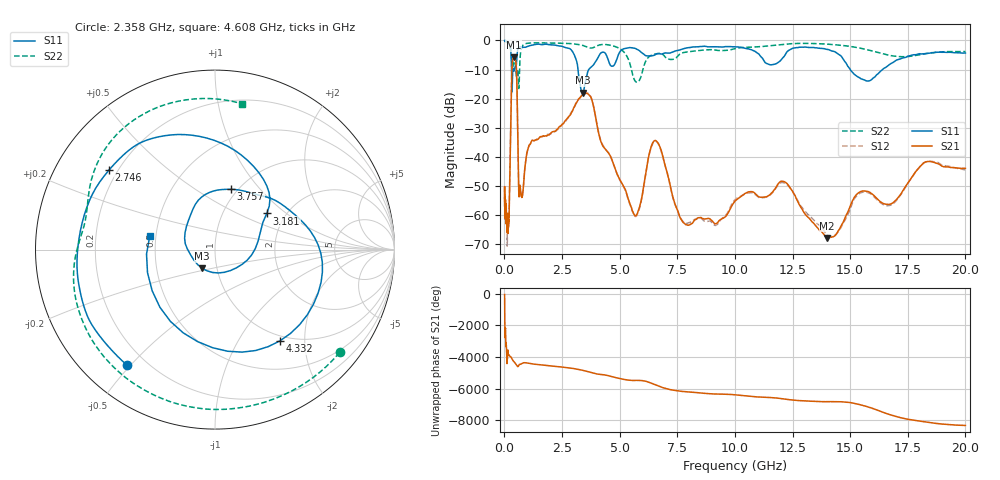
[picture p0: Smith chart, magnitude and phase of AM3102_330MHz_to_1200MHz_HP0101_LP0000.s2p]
! Date/Time: Tue, Sep 11, 2018 5:13 PM
! Network Analyzer: Agilent Technologies E8362B Rev: A.07.50.63
! Sweep from 0.010 to 20.000 GHz, 1601 Points, Sweep Type: LOG
! Power Supply: 4.949 V, 0.001 A
# Hz S DB R 50
!freq MagS11 AngS11 MagS21 AngS21 MagS12 AngS12 MagS22 AngS22
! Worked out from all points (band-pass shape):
!   1601 points, 10 MHz to 20 GHz, reference 50 ohm
!   highest |S21| = -5.85 dB at 412.5 MHz (marker M1); lowest = -67.9 dB at 14.01 GHz (marker M2)
!   |S21| within 3 dB of the highest: 332.1 MHz to 515.1 MHz (182.9 MHz wide, 43.2 % of centre)
!   lowest |S11| = -18.0 dB at 3.4 GHz (marker M3), VSWR 1.29, Z = 42.4 - j8.97 ohm
!   |S11| at or under -10 dB: 309.7 MHz to 367.7 MHz (57.91 MHz wide, 17.1 % of centre); 3.193 GHz to 3.661 GHz (468.2 MHz wide, 13.7 % of centre); 15.01 GHz to 16.41 GHz (1.4 GHz wide, 8.91 % of centre)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
!   |S22| runs from -16.5 to -0.2 dB; largest |S21 - S12| = 0.0063
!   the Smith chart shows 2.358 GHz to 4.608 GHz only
!   S11 on the Smith chart (normalised r, x): 2.358 GHz: 0.13, -0.49; 2.746 GHz: 0.17, +0.32; 3.181 GHz: 1.60, +0.74; 3.757 GHz: 0.93, +0.71; 4.332 GHz: 0.92, -1.53; 4.608 GHz: 0.46, +0.08
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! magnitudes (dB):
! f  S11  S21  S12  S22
! 10 MHz  0.0  -57.0  -50.5  -0.2
! 35.55 MHz  0.0  -59.9  -59.3  -0.3
! 126.4 MHz  -0.4  -65.5  -69.6  -0.7
! 208.1 MHz  -1.3  -58.9  -59.1  -1.4
! 412.5 MHz  -10.5  -5.8  -5.9  -7.3
! 447.2 MHz  -9.5  -6.1  -6.1  -7.3
! 530.6 MHz  -7.3  -11.6  -11.6  -12.5
! 635.6 MHz  -2.3  -53.7  -53.4  -15.9
! 1.59 GHz  -1.4  -33.1  -33.1  -0.8
! 2.358 GHz  -1.8  -29.9  -30.2  -0.9
! 2.746 GHz  -2.6  -26.7  -26.8  -1.0
! 3.181 GHz  -9.1  -20.6  -20.8  -1.3
! 3.4 GHz  -18.0  -18.5  -18.7  -1.7
! 3.757 GHz  -9.2  -19.6  -19.5  -2.6
! 4.332 GHz  -4.1  -36.9  -36.8  -1.4
! 4.608 GHz  -8.6  -39.9  -40.0  -1.7
! 5.652 GHz  -2.7  -60.1  -60.4  -13.7
! 6.58 GHz  -4.7  -34.5  -34.7  -4.6
! 7.845 GHz  -2.7  -63.2  -62.8  -4.0
! 12.09 GHz  -5.9  -48.5  -48.9  -1.4
! 14.01 GHz  -3.1  -67.9  -67.1  -1.3
! 20 GHz  -4.3  -44.0  -44.5  -3.8
